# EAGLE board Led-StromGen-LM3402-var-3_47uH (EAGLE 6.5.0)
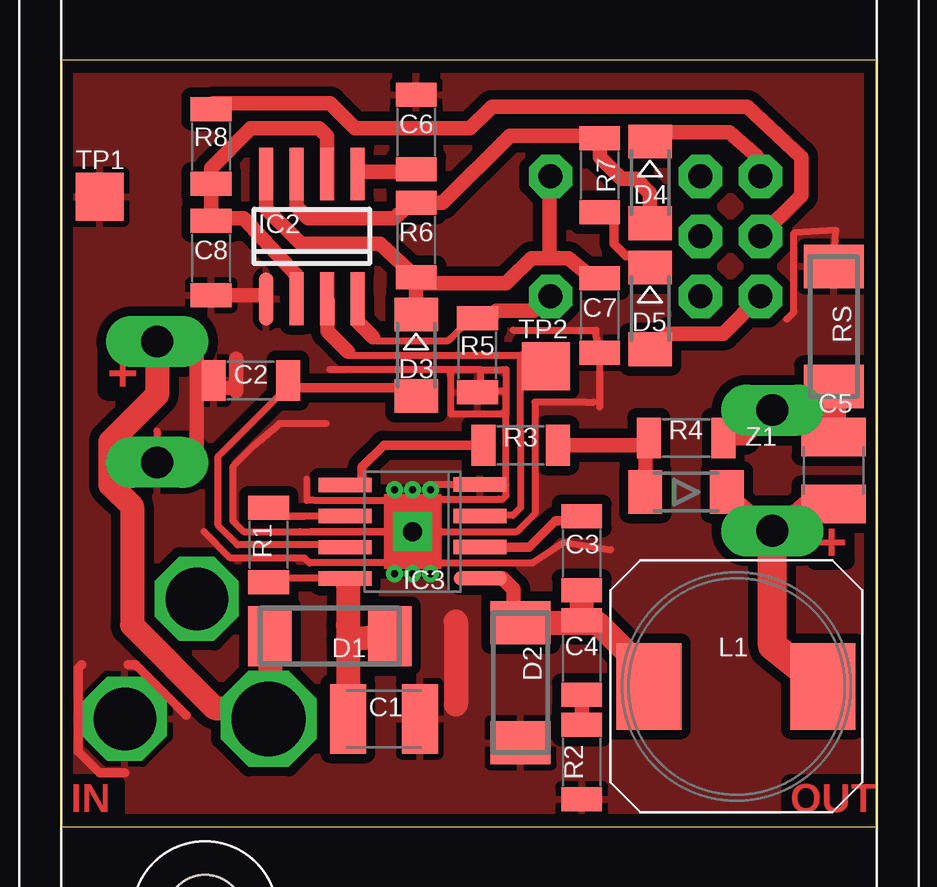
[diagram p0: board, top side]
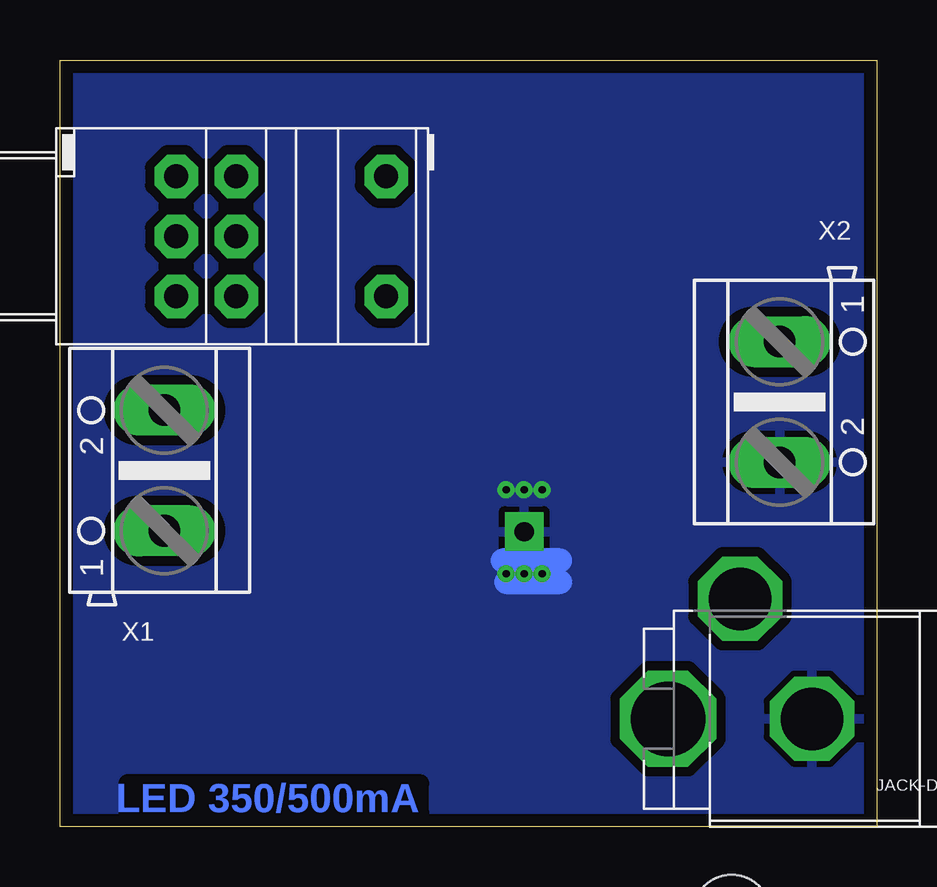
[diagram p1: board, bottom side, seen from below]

Size 34.05 x 31.95 mm. Coordinates in mm from the lower left corner, seen from the top.
Outline: 0,31.95 0,0 34.05,0 34.05,31.95 0,31.95
Copper layers ((1*2)+(15*16)): Top 0.035mm / dielectric 0.7mm / Route2 0.035mm / dielectric 0.15mm / Route15 0.035mm / dielectric 0.7mm / Bottom 0.035mm
Design rules "default *": minimum track width 0.3mm, minimum drill 0.3mm, track to track 0.15mm, track to pad 0.15mm, pad to pad 0.15mm, via to via 0.15mm, smd to smd 2mil, copper to edge 20mil, drill to drill 7mil, minimum pad ring 16mil, minimum via ring 8mil, stop-mask expansion 0.05mm, vias tented up to drill 0.6mm, thermal gap 10mil

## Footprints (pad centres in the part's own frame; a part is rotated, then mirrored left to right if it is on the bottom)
STRAPUBOX-2090 = hole 3.2: 9,31; 120,9
C1210K = smd 1.5 x 2.9: 1 -1.5,0; 2 1.5,0
C1206 = smd 1 x 1.7: 1 -1.55,0; 2 1.55,0
C1210 = smd 1.6 x 2.7: 1 -1.4,0; 2 1.4,0
MINI_MELF-0207R = smd 1.8 x 2.5: 1 -2.5,0; 2 2.5,0
MINIMELF = smd 1.4 x 1.8: A 1.7,0; C -1.7,0
SO08 = smd 0.6 x 2.2: 1 -1.905,-2.6; 2 -0.635,-2.6; 3 0.635,-2.6; 4 1.905,-2.6; 5 1.905,2.6; 6 0.635,2.6; 7 -0.635,2.6; 8 -1.905,2.6
MSOP8 = smd 0.6 x 2.2: 1 -1.948,-2.815; 2 -0.647,-2.812; 3 0.65,-2.812; 4 1.955,-2.812; 5 1.95,2.812; 6 0.645,2.812; 7 -0.65,2.817; 8 -1.948,2.817 | drill 0.8 square: DAB 0,0
JACK-DC_10 = drill 3.1 octagon: PIN 6,0 | drill 2.6 octagon: SLIDE 0,0; SW 3,-5
B82464... = smd 3.6 x 2.7: 1 0,3.65; 2 0,-3.6
P092S = drill 1 octagon: A1 -5,-2.5; A2 -7.5,-2.5; E1 -5,2.5; E2 -7.5,2.5; S1 -5,0; S2 -7.5,0; SW -13.75,2.5; SW1 -13.75,-2.5
1206 = smd 1 x 1.7: 1 -1.55,0; 2 1.55,0
TP20SQ = smd 2 x 2: TP 0,0
AK500/2 = drill 1.321 long: 1 -2.515,0; 2 2.515,0
MELF-LM34 = smd 1.4 x 1.8: 1 -1.7,0; 2 1.7,0

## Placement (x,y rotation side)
BOX1  STRAPUBOX-2090; hier können bis zu 3 Leiterplatten eingebaut werden, z.B. für RGB, wobei der Anschlussstecker für Power nur auf einer einzigen bestückt wird. Die interne Verbindung für Power erfolgt dann über die Klemme X2.  [STRAPUBOX-2090]  37.05,-12.6 90 top
C1  4μ7 50V  [C1210K]  13.5,4.5 0 top
C2  1μ  [C1206]  7.95,18.6 180 top
C3  10n  [C1206]  21.75,11.4 270 top
C4  100n  [C1206]  21.75,7.05 270 top
C5  1μ 100V  [C1210]  32.25,14.85 90 top
C6  10n  [C1206]  14.85,28.95 90 top
C7  100n  [C1206]  22.5,21.3 270 top
C8  33n  [C1206]  6.3,23.7 270 top
D1  SMS1100  [MINI_MELF-0207R]  11.25,7.95 180 top
D2  SMS1100  [MINI_MELF-0207R]  19.2,6 270 top
D3  LL4148  [MINIMELF]  14.85,19.65 270 top
D4  LL4148  [MINIMELF]  24.6,26.85 270 top
D5  LL4148  [MINIMELF]  24.6,21.6 270 top
IC2  ICM7555CD  [SO08]  10.5,24.6 0 top
IC3  LM3402  [MSOP8]  14.7,12.3 90 top
J2  JACK-DC_10  [JACK-DC_10]  2.7,4.5 180 bottom
L1  47μH  [B82464...]  28.2,5.85 90 top
P1  P092S  [P092S]  34.2,24.6 180 bottom
R1  220k  [1206]  8.7,11.75 270 top
R2  22R  [1206]  21.75,2.7 90 top
R3  0R  [1206]  19.2,15.9 180 top
R4  1k  [1206]  26.1,16.2 180 top
R5  82k  [1206]  17.4,19.65 90 top
R6  4k7  [1206]  14.85,24.45 270 top
R7  100R  [1206]  22.5,27.15 90 top
R8  4k7  [1206]  6.3,28.35 90 top
RS  0R68  [MINI_MELF-0207R]  32.25,20.85 270 top
TP1  GND  [TP20SQ]  1.65,26.25 0 top
TP2  PWM  [TP20SQ]  20.25,19.2 0 top
X1  [AK500/2]  29.7,14.85 90 bottom
X2  [AK500/2]  4.05,17.7 270 bottom
Z1  39V  [MELF-LM34]  26.1,13.95 180 top

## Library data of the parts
BOX1 = Enclosures-DIN-Rail+more_1
C1 = rcl; OPTION: bis 50V
C2-C8 R1-R8 RS = rcl
D1 D2 IC3 = LED-Treiber
D3-D5 = SMD-rcldf_led
IC2 = linear
J2 = allgem
L1 = inductor-fastron; BUERKLIN-73D90--: 1uH bis 1000uH
P1 = pot
TP1 TP2 = testpad
X1 X2 = con-ptr500
Z1 = allgem; BUERKLIN-25S7360: 500mW mini-MELF

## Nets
7V: C7.1 D3.C IC2.8 P1.SW1 R6.2
GND: C1.2 C2.2 C6.2 C7.2 C8.2 D2.2 IC2.1 IC3.4 IC3.DAB J2.SLIDE R2.1 R5.1 RS.1 TP1.TP X2.2
N$1: IC3.5 R3.2
N$2: C4.2 R2.2
N$3: C3.2 C4.1 D2.1 IC3.1 L1.1
N$4: IC3.6 R1.1
N$5: C5.1 L1.2 X1.1 Z1.1
N$6: C5.2 R4.1 RS.2 X1.2
N$7: D1.2 J2.PIN X2.1
N$8: C3.1 IC3.2
N$9: C2.1 D3.A IC3.7
N$10: R3.1 R4.2 Z1.2
N$11: P1.S1 R8.2
N$13: C8.1 IC2.2 IC2.6 R8.1
N$14: C6.1 IC2.5
N$20: D4.A IC2.7 R6.1 R7.2
N$22: D5.A P1.E1
N$33: D4.C P1.A1
N$53: D5.C R7.1
ON-OFF: IC2.4 P1.SW R5.2
PWM: IC2.3 IC3.3 TP2.TP
VIN+: C1.1 D1.1 IC3.8 R1.2

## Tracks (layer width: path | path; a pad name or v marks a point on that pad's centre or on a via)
7V
  Top 0.6: IC2.8 8.6,25.75 10.05,24.3 13.35,24.3 R6.2 | R6.2 D3.C | P1.SW1 20.45,26.95 20.4,26.4 20.4,23.7 | 20.4,23.7 21.2,23.7 21.9,23.1 22.45,22.85 C7.1 | 20.4,23.7 19.65,23.7 18.7,22.75 18.6,22.65 15.1,22.65 R6.2
GND  (via drill 0.3)
  Top 0.3: 19.8,13.05 19.8,17.7 21.9,17.7 22.25,17.7 | 19.8,13.05 19.05,12.3 | 19.05,12.3 19.8,13.05 | 7.2,18.3 5.85,18.25 7.35,18.3 7.35,18.15 7.35,19.5 | 15.9,12.3 19.05,12.3 | 30.3,21.15 30.6,21.45 30.6,24.75 32.35,24.85 RS.1 | 15.75,13.65 18.3,13.65 18.45,13.65 18.6,13.8 18.6,14.25 18.6,17.2 | 18.6,17.2 18.6,18.15 | 11.1,16.8 9.15,16.8 8.1,15.9 7.2,15 7.2,12.75 7.65,12.3 10,12.3 10.45,12.3 | 10.45,12.3 13.5,12.3 10.45,12.3 | 15.95,11 19.7,11 21,11.85 22.95,11.55 | 18.6,18.15 17.55,18.15 | 17.55,18.15 R5.1 17.55,18.15 | 17.55,18.15 17.55,19.05 | 17.55,19.05 16.3,19.05 | 16.3,19.05 11.25,19.05 | 4.05,16.5 4.05,15.15 | 17.55,19.05 18.45,19.05 18.6,19.05 18.6,18.15 | 18.6,18.15 18.6,17.2 | 18.6,17.2 16.3,17.2 16.3,19.05 | 6,12.3 7.1,11.2 10.2,11.2 10.4,11 13.6,11 13.95,10.65 v13.95,10.55 | 10.3,14.5 10.3,13.6 10.6,13.6 13.65,13.6 13.95,13.9 v13.95,14.05 | 18.9,20.7 22.35,20.7 22.35,20.5 C7.2 22.5,17.5 | IC3.4 15.65,14.26 v15.45,14.05
  Top 0.4: 2.85,6.75 3.15,6.75 5.25,4.65 | 0.9,6.75 0.75,6.6 0.75,3.15 1.65,2.25 2.7,2.25
  Top 0.6: C8.2 8.45,22.15 8.55,22.05 IC2.1 | 7.2,18.3 7.35,18.3 | 7.35,18.3 7.35,18.15 | 7.35,18.15 7.35,19.5 | 7.35,19.5 7.35,18.15 | 7.35,18.15 7.35,19.5 | 7.35,19.5 7.35,18.15 | 7.35,18.15 7.35,18.3 | 7.35,18.3 5.85,18.25 C2.2 | 4.05,15.15 5.7,15.15 5.7,19.5
  Top 1: 16.5,8.55 16.5,5.1
  Bottom 1: 13.2,11.1 15.6,11.1 13.65,10.65 | 13.65,10.65 15.45,10.2 13.2,10.2 14.25,10.65 13.65,10.65
  other vias: 14.7,14.05 14.7,10.55 15.45,10.55
  pour Top (isolate 0.4): 33.75,0.15 33.75,31.65 0.3,31.65 0.15,0.15
  pour Bottom (isolate 0.4): 34.65,31.5 34.5,0.3 0.3,0.3 0.3,31.5
N$1
  Top 0.4: 12.3,14.25 12.6,14.4 12.6,15 13.5,15.9 R3.2
  Top 0.6: IC3.5 12.3,14.25
N$2
  Top 0.6: C4.2 R2.2
N$3
  Top 0.3: C4.1 21.75,8.65 21.9,8.5
  Top 0.6: IC3.1 18.45,10.35 18.9,9.9 18.9,8.95 D2.1
  Top 1: C4.1 C3.2 | D2.1 21.9,8.5 22.4,8.5 24,6.9 24,6.4 L1.1
N$4
  Top 0.3: IC3.6 10.21,12.95 | 10.21,12.95 9.26,12.95 | 9.26,12.95 10.21,12.95 | 10.21,12.95 9.26,12.95 | 9.26,12.95 10.21,12.95 | 10.21,12.95 9.26,12.95 | 9.26,12.95 9.15,13.05 R1.1
N$5
  Top 0.6: 29.64,12.34 Z1.1
  Top 1: X1.1 29.64,12.34
  Top 1.2: L1.2 29.7,7.54 X1.1 30.18,12.34 31.35,13.35 32.15,13.35 C5.1
N$6
  Top 0.6: R4.1 28.54,16.2 X1.2
  Top 1: RS.2 32.25,17.25 | 32.25,17.25 C5.2 | X1.2 32.13,17.36 32.25,17.25
N$7
  Top 1: X2.1 4.05,18 2.1,16.05 2.1,14.25 3,13.35 3,8.4 6.45,4.95 8.25,4.95 J2.PIN 8.75,4.55 D1.2
N$8
  Top 0.4: IC3.2 19.55,11.65 20.65,12.75 21.25,12.75 C3.1
N$9
  Top 0.3: 9.45,18.3 9.6,18.15 | 9.6,18.15 9.35,18.3 9.45,18.15 | 9.45,18.15 9.45,18.25 | 9.45,18.25 C2.1 | 9.45,18.25 9.45,18.15 | 9.45,18.15 9.6,18.15 | 9.6,18.15 9.45,18.3 | 14.25,18.3 14.4,17.85 14.65,18 D3.A | IC3.7 11.4,11.7 11.1,11.7 10.9,11.75 7.4,11.75 6.6,12.55 6.6,15.45 9.45,18.3
  Top 0.4: 9.45,18.3 14.25,18.3
N$10
  Top 0.6: R3.1 20.8,15.9 24.3,15.9 R4.2 24.4,15.3 Z1.2
N$11
  Top 0.6: R8.2 6.4,30.15 11.25,30.15 12.3,29.1 17.1,29.1 17.93,29.93 18,30 28.65,30 30.9,27.9 30.9,26.3 P1.S1
N$13
  Top 0.6: IC2.6 11.13,28.77 10.8,29.1 8.15,29.1 7.95,29.1 6.3,27.45 R8.1 C8.1 5.75,25.35 7.65,25.35 9.87,22.98 IC2.2
N$14
  Top 0.6: IC2.5 12.4,27.7 12.45,27.3 14.8,27.3 C6.1
N$20
  Top 0.6: IC2.7 9.87,25.84 10.35,25.35 13.95,25.35 | 13.95,25.35 14.4,25.8 | 14.4,25.8 R6.1 15.95,26 18.75,28.8 22.1,28.8 R7.2 22.5,27.9 23.4,27 24,27 24.6,26.4 D4.A | 14.4,25.8 13.95,25.35
N$22
  Top 0.6: D5.A 25.3,20.5 25.35,20.55 27.65,20.55 P1.E1
N$33
  Top 0.6: P1.A1 29.05,27.95 27.9,28.95 24.85,28.95 D4.C
N$53
  Top 0.3: D5.C 23.95,23.8
  Top 0.4: 22.7,25.75 22.95,25.65 23.1,25.5 23.1,24.3 23.6,23.8 23.95,23.8
  Top 0.6: R7.1 22.7,25.75
ON-OFF
  Top 0.3: 13.05,20.4 13.2,20.25 16.15,20.25 16.35,20.4 17.1,21.15 R5.2
  Top 0.6: IC2.4 12.4,21.05 13.05,20.4 | P1.SW 20.4,22.05 19.75,21.5 18.2,21.5 18,21.3 R5.2
PWM
  Top 0.3: IC2.3 11.1,22.04 | 19.2,19.65 12,19.65 12,19.8 11.88,19.91 11.7,20.1 | 19.2,19.65 19.35,19.65 19.2,19.65 | 19.2,19.65 19.2,16.5 19.2,16.2 19.2,13.3 18.88,12.98 17.24,12.98 IC3.3 | 19.2,19.65 19.5,19.05 TP2.TP
  Top 0.6: IC2.3 11.15,21.91 11.15,20.65 11.7,20.1 11.88,19.91 | 11.88,19.91 12,19.8 11.88,19.91
VIN+
  Top 0.3: IC3.8 9.05,10.35 R1.2
  Top 0.6: IC3.8 12.15,9.9 12,10.05 | 12,5.1 C1.1
  Top 1: 12,10.05 12,8.4 12,7.8 | 12,7.8 12,5.1 | D1.1 12,7.8

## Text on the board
Top: + | + | IN | OUT
Bottom: LED 350/500mA
Reference: PCB: 34x32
